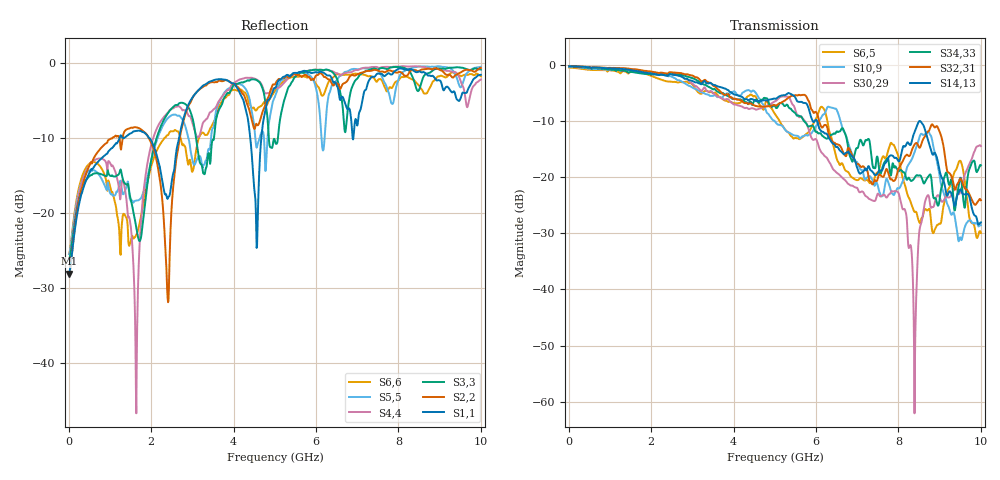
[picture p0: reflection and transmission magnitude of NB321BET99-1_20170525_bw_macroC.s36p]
! Touchstone(R) file created by SIwave 2017.0.0
! Touchstone(R) file created on Mon Jun 05 09:02:04 2017
! Port[1] = D_CN_0__DIE_137
! Port[2] = D_CN_0__LGA_AL5
! Port[3] = D_CN_1__DIE_141
! Port[4] = D_CN_1__LGA_AF2
! Port[5] = D_CN_2__DIE_145
! Port[6] = D_CN_2__LGA_AE1
! Port[7] = D_CN_3__DIE_151
! Port[8] = D_CN_3__LGA_AB2
! Port[9] = D_CN_4__DIE_161
! Port[10] = D_CN_4__LGA_AL9
! Port[11] = D_CN_5__DIE_167
! Port[12] = D_CN_5__LGA_AK14
! Port[13] = D_CN_6__DIE_171
! Port[14] = D_CN_6__LGA_AL17
! Port[15] = D_CN_7__DIE_175
! Port[16] = D_CN_7__LGA_AL21
! Port[17] = D_CP_0__DIE_138
! Port[18] = D_CP_0__LGA_AL7
! Port[19] = D_CP_1__DIE_142
! Port[20] = D_CP_1__LGA_AG1
! Port[21] = D_CP_2__DIE_146
! Port[22] = D_CP_2__LGA_AC1
! Port[23] = D_CP_3__DIE_152
! Port[24] = D_CP_3__LGA_AA1
! Port[25] = D_CP_4__DIE_162
! Port[26] = D_CP_4__LGA_AK10
! Port[27] = D_CP_5__DIE_168
! Port[28] = D_CP_5__LGA_AL15
! Port[29] = D_CP_6__DIE_172
! Port[30] = D_CP_6__LGA_AK18
! Port[31] = D_CP_7__DIE_176
! Port[32] = D_CP_7__LGA_AL19
! Port[33] = DCLK_CN_DIE_156
! Port[34] = DCLK_CN_LGA_AL11
! Port[35] = DCLK_CP_DIE_157
! Port[36] = DCLK_CP_LGA_AL13
! S-parameters (magnitude in dB)
# Hz S DB R 50.000000
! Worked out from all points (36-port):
!   1000 points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, 10 MHz to 10 GHz, reference 50 ohm
!   strongest paths, dB at 10 MHz, 2.51 GHz, 5.01 GHz, 7.51 GHz, 10 GHz:
!     S14,13: -0.2, -1.7, -6.0, -19.1, -28.1
!     S32,31: -0.2, -1.3, -7.2, -19.9, -24.1
!     S34,33: -0.3, -1.7, -7.4, -17.3, -17.9
!     S30,29: -0.2, -1.5, -6.5, -22.9, -14.5
!     S10,9: -0.3, -2.1, -10.1, -21.9, -28.6
!     S6,5: -0.5, -3.0, -8.8, -19.1, -29.9
!   lowest |S11| = -28.1 dB at 10 MHz (marker M1), VSWR 1.08, Z = 54.1 + j0.46 ohm
!   |S11| at or under -10 dB: start of sweep to 1.234 GHz; 1.957 GHz to 2.676 GHz (718.8 MHz wide, 31 % of centre); 4.405 GHz to 4.673 GHz (267.6 MHz wide, 5.9 % of centre)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
